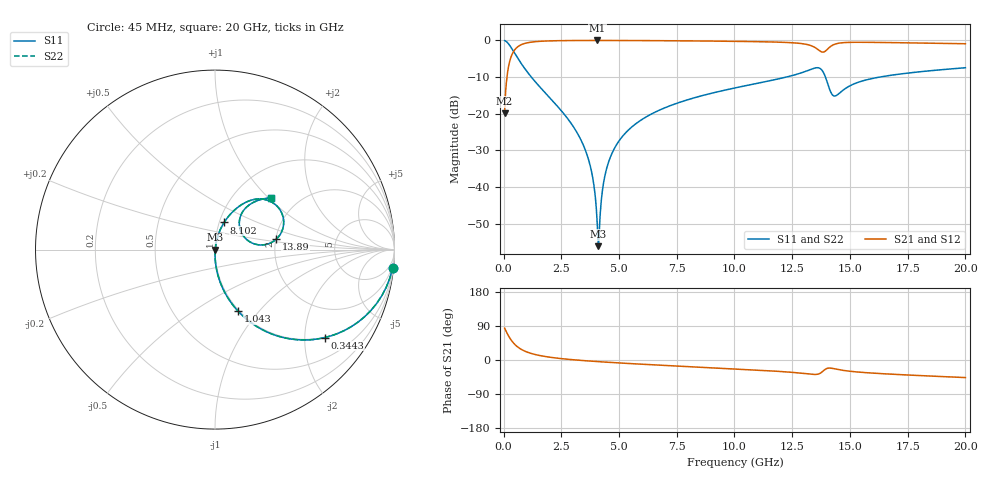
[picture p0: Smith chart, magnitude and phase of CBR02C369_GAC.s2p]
! S-parameter model data by Modelithics Inc.  support@modelithics.com 813-866-6335  Tampa FL USA
! S-Parameter data specifications:
! Substrate: 20-mil Rogers 4350B, substrate thickness, H=0.508mm, Dielectric constant, Er=3.75
! PCB Mounting Pad Footprint: Pad width, PadW=0.32mm , Pad length, PadL=0.37mm , Pad gap, PadG (edge-to-edge)=0.19mm , Reference planes=0.93mm apart
#  GHz  S  MA  R 50
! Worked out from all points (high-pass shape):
!   801 points, 45 MHz to 20 GHz, reference 50 ohm
!   highest |S21| = -0.01 dB at 4.061 GHz (marker M1); lowest = -19.8 dB at 45 MHz (marker M2)
!   |S21| within 3 dB of the highest: 434.4 MHz to 13.73 GHz (13.3 GHz wide, 188 % of centre); 13.91 GHz to end of sweep
!   lowest |S11| = -56.1 dB at 4.111 GHz (marker M3), VSWR 1.00, Z = 50.2 + j0.00115 ohm
!   |S11| at or under -10 dB: 1.203 GHz to 12.24 GHz (11.04 GHz wide, 164 % of centre); 13.94 GHz to 16.28 GHz (2.343 GHz wide, 15.5 % of centre)
!   |S22| runs from -56.1 to 0.0 dB; largest |S21 - S12| = 0
!   S11 on the Smith chart (normalised r, x): 45 MHz: 1, -19; 344.3 MHz: 0.99, -2.51; 1.043 GHz: 0.99, -0.78; 8.102 GHz: 1.05, +0.33; 13.89 GHz: 2.01, +0.27; 20 GHz: 1.47, +1.03
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0.045  0.9948 -5.9  0.102 84.1  0.102 84.1  0.9948 -5.9
0.194662  0.9137 -24.2  0.4061 65.8  0.4061 65.8  0.9137 -24.2
0.344325  0.7844 -38.7  0.6197 51.3  0.6197 51.3  0.7844 -38.7
0.64365  0.5535 -57.0  0.832 32.9  0.832 32.9  0.5535 -57.0
1.04275  0.3662 -69.5  0.9295 20.4  0.9295 20.4  0.3662 -69.5
3.387462  0.04163 -89.2  0.9976 -1.2  0.9976 -1.2  0.04163 -89.2
3.811506  0.01619 -87.7  0.9983 -3.1  0.9983 -3.1  0.01619 -87.7
4.060944  0.002939 -62.2  0.9984 -4.2  0.9984 -4.2  0.002939 -62.2
4.110831  0.001567 0.4  0.9984 -4.4  0.9984 -4.4  0.001567 0.4
4.185663  0.004307 63.9  0.9983 -4.7  0.9983 -4.7  0.004307 63.9
4.285437  0.009219 75.0  0.9983 -5.1  0.9983 -5.1  0.009219 75.0
4.410156  0.01535 78.5  0.9982 -5.6  0.9982 -5.6  0.01535 78.5
4.784313  0.03299 80.2  0.9977 -7.0  0.9977 -7.0  0.03299 80.2
5.532625  0.06524 78.9  0.996 -9.6  0.996 -9.6  0.06524 78.9
6.704981  0.1104 75.6  0.9919 -13.5  0.9919 -13.5  0.1104 75.6
8.101831  0.1597 71.5  0.9849 -17.8  0.9849 -17.8  0.1597 71.5
10.0225  0.2251 65.6  0.9712 -23.6  0.9712 -23.6  0.2251 65.6
13.36496  0.4091 41.0  0.8366 -37.8  0.8366 -37.8  0.4091 41.0
13.88878  0.3462 9.6  0.6991 -26.5  0.6991 -26.5  0.3462 9.6
14.33777  0.1745 30.1  0.8858 -23.3  0.8858 -23.3  0.1745 30.1
16.68248  0.3315 51.4  0.9344 -37.1  0.9344 -37.1  0.3315 51.4
20  0.4238 43.0  0.9006 -46.4  0.9006 -46.4  0.4238 43.0
